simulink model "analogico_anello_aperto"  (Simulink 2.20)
settings: Solver=ode45  StartTime=0.0  StopTime=10.0  RelTol=1e-3  AbsTol=1e-6

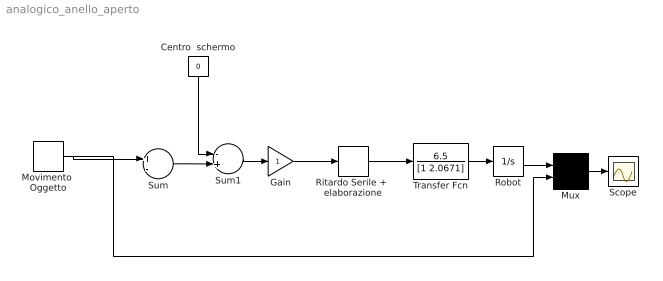
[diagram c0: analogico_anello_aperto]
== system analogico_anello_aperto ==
  Centro  schermo : Constant  Orientation=down  Value=0
  Gain : Gain  Gain=1
  Movimento  Oggetto : DiscretePulseGenerator  Amplitude=1  Period=100  PulseWidth=10  PhaseDelay=10  SampleTime=.1
  Mux : Mux  Inputs=2
  Ritardo Serile +  elaborazione : TransportDelay  DelayTime=.190  InitialInput=0  BufferSize=1024
  Robot : Integrator  ExternalReset=none  InitialConditionSource=internal  InitialCondition=0  LimitOutput=off  UpperSaturationLimit=inf  LowerSaturationLimit=-inf  ShowSaturationPort=off  ShowStatePort=off  AbsoluteTolerance=auto
  Scope : Scope
  Sum : Sum  Inputs=+-
  Sum1 : Sum  Inputs=-+
  Transfer Fcn : TransferFcn  Numerator=6.5  Denominator=[1 2.0671]
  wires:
  Movimento  Oggetto/1 -> Sum/1, Mux/2
  Mux/1 -> Scope/1
  Sum/1 -> Sum1/2
  Centro  schermo/1 -> Sum1/1
  Gain/1 -> Ritardo Serile +  elaborazione/1
  Sum1/1 -> Gain/1
  Transfer Fcn/1 -> Robot/1
  Robot/1 -> Mux/1
  Ritardo Serile +  elaborazione/1 -> Transfer Fcn/1
